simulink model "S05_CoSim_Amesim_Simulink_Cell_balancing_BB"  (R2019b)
settings: Solver=ode23s  StartTime=0  StopTime=25000  FixedStep=0.5  RelTol=1e-3  EnableMultiTasking=on
undefined symbols (not defined in the file): S05_CoSim_Amesim_Simulink_Cell_balancing
libraries: simulink x1
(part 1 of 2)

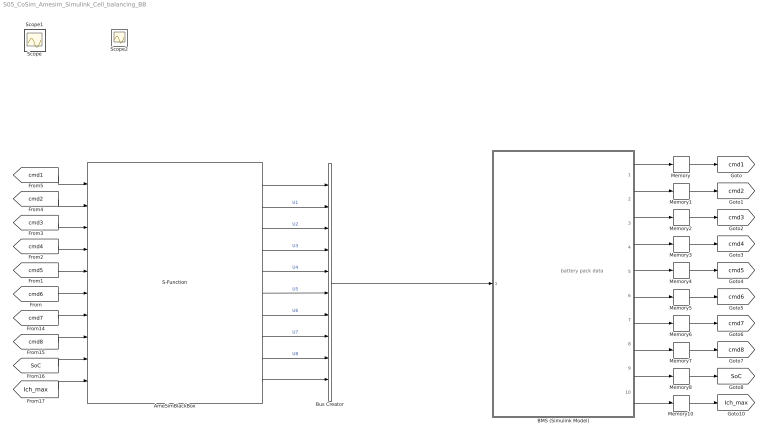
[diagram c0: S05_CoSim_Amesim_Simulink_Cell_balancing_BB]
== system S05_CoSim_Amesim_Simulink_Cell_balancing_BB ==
  note: battery pack data
  " BMS (Simulink Model)" : Subsystem
  AmeSimBlackBox : S-Function  InitFcn=clear S05_CoSim_Amesim_Simulink_Cell_balancing  StopFcn=clear S05_CoSim_Amesim_Simulink_Cell_balancing  FunctionName=S05_CoSim_Amesim_Simulink_Cell_balancing  Parameters=[0 0.01] [allrealparamnames] [allrealparamvalues] [allintparamnames] [allintparamvalues] [alltxtparamnames] [alltxtparamvalues]  SFunctionDeploymentMode=off  EnableBusSupport=off  mask(Simcenter Amesim S-function: S05_CoSim_Amesim_Simulink_Cell_balancing){IL_ns_paths=4, IL_SOCinit=90, IL_Cn=42, IL_Ichbalancing=8, IL_Idchbalancing=-8, IL_Tinit=23, IL_Tamb=23, IL_h_cell=222, IL_w_cell=211, IL_t_cell=12, IL_t_plate=1.5, IL_t_path=0.8, IL_w_path=2, IL_l_path=222, IL_DSOC1=3.46, IL_DSOC2=-4.33, IL_DSOC3=0.5, IL_DSOC4=0.38, IL_DSOC5=4.63, IL_DSOC6=-0.77, IL_DSOC7=2.73, IL_DSOC8=-1.36, IL_Ccoef1=1.033, IL_Ccoef2=1.053, IL_Ccoef3=0.953, IL_Ccoef4=1.058, IL_Ccoef5=0.926, IL_Ccoef6=1.064, IL_Ccoef7=0.956, IL_Ccoef8=1.077, IL_Rcoef1=0.93, IL_Rcoef2=0.876, IL_Rcoef3=1.029, IL_Rcoef4=0.863, IL_Rcoef5=0.85, IL_Rcoef6=1.044, IL_Rcoef7=0.878, IL_Rcoef8=1.146}
      mask prompts: IL_ns_paths "number of path per plate"; IL_SOCinit "inital state of charge"; IL_Cn "nominal capacity"; IL_Ichbalancing "balancing charge current"; IL_Idchbalancing "balancing discharge current"; IL_Tinit "initial temperature"; IL_Tamb "ambiant temperature"; IL_h_cell "height of the cell"; IL_w_cell "width of the cell"; IL_t_cell "thickness of the cell"; IL_t_plate "thickness of the plate"; IL_t_path "thickness of the coolant path"; IL_w_path "width of the coolant path"; IL_l_path "length of the coolant path"; IL_DSOC1 "SOC dispersion - cell 1"; IL_DSOC2 "SOC dispersion - cell 2"; IL_DSOC3 "SOC dispersion - cell 3"; IL_DSOC4 "SOC dispersion - cell 4"; IL_DSOC5 "SOC dispersion - cell 5"; IL_DSOC6 "SOC dispersion - cell 6"; IL_DSOC7 "SOC dispersion - cell 7"; IL_DSOC8 "SOC dispersion - cell 8"; IL_Ccoef1 "capacity dispersion coefficient - cell 1"; IL_Ccoef2 "capacity dispersion coefficient - cell 2"; IL_Ccoef3 "capacity dispersion coefficient - cell 3"; IL_Ccoef4 "capacity dispersion coefficient - cell 4"; IL_Ccoef5 "capacity dispersion coefficient - cell 5"; IL_Ccoef6 "capacity dispersion coefficient - cell 6"; IL_Ccoef7 "capacity dispersion coefficient - cell 7"; IL_Ccoef8 "capacity dispersion coefficient - cell 8"; IL_Rcoef1 "resistance dispersion coefficient - cell 1"; IL_Rcoef2 "resistance dispersion coefficient - cell 2"; IL_Rcoef3 "resistance dispersion coefficient - cell 3"; IL_Rcoef4 "resistance dispersion coefficient - cell 4"; IL_Rcoef5 "resistance dispersion coefficient - cell 5"; IL_Rcoef6 "resistance dispersion coefficient - cell 6"; IL_Rcoef7 "resistance dispersion coefficient- cell 7"; IL_Rcoef8 "resistance dispersion coefficient - cell 8"
      mask help: Mask for Simcenter Amesim to Simulink black-box.
      mask init:
      | allintparamnames=strvcat('ns_paths');allintparamvalues=[IL_ns_paths];allrealparamnames=strvcat('SOCinit','Cn','Ichbalancing','Idchbalancing','Tinit','Tamb','h_cell','w_cell','t_cell','t_plate','t_path','w_path','l_path','DSOC1','DSOC2','DSOC3','DSOC4','DSOC5','DSOC6','DSOC7','DSOC8','Ccoef1','Ccoef2','Ccoef3','Ccoef4','Ccoef5','Ccoef6','Ccoef7','Ccoef8','Rcoef1','Rcoef2','Rcoef3','Rcoef4','Rcoef5','Rcoef6','Rcoef7','Rcoef8');allrealparamvalues=[IL_SOCinit;IL_Cn;IL_Ichbalancing;IL_Idchbalancing;IL_Tinit;IL_Tamb;IL_h_cell;IL_w_cell;IL_t_cell;IL_t_plate;IL_t_path;IL_w_path;IL_l_path;IL_DSOC1;IL_DSOC2;IL_DSOC3;IL_DSOC4;IL_DSOC5;IL_DSOC6;IL_DSOC7;IL_DSOC8;IL_Ccoef1;IL_Ccoef2;IL_Ccoef3;IL_Ccoef4;IL_Ccoef5;IL_Ccoef6;IL_Ccoef7;IL_Ccoef8;IL_Rcoef1;IL_Rcoef2;IL_Rcoef3;IL_Rcoef4;IL_Rcoef5;IL_Rcoef6;IL_Rcoef7;IL_Rcoef8];alltxtparamnames=[];alltxtparamvalues=[];
  Bus Creator : BusCreator  Inputs=10
  Memory{,1..8,10} (10 alike) : Memory
  Scope : Scope
  Scope1 : Scope
  Scope2 : Scope
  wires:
  Memory/1 -> [cmd1]
  Memory2/1 -> [cmd3]
  Memory4/1 -> [cmd5]
  Memory3/1 -> [cmd4]
  Memory1/1 -> [cmd2]
  Memory5/1 -> [cmd6]
  Memory6/1 -> [cmd7]
  Memory7/1 -> [cmd8]
  Memory8/1 -> [SoC]
  AmeSimBlackBox/10 -> Bus Creator/10  "T"
  AmeSimBlackBox/9 -> Bus Creator/9  "U8"
  AmeSimBlackBox/7 -> Bus Creator/7  "U6"
  AmeSimBlackBox/6 -> Bus Creator/6  "U5"
  AmeSimBlackBox/5 -> Bus Creator/5  "U4"
  AmeSimBlackBox/4 -> Bus Creator/4  "U3"
  AmeSimBlackBox/3 -> Bus Creator/3  "U2"
  AmeSimBlackBox/2 -> Bus Creator/2  "U1"
  AmeSimBlackBox/8 -> Bus Creator/8  "U7"
  [cmd1] -> AmeSimBlackBox/1
  [cmd2] -> AmeSimBlackBox/2
  [cmd3] -> AmeSimBlackBox/3
  [cmd4] -> AmeSimBlackBox/4
  [cmd5] -> AmeSimBlackBox/5
  [cmd6] -> AmeSimBlackBox/6
  [cmd7] -> AmeSimBlackBox/7
  [cmd8] -> AmeSimBlackBox/8
  [SoC] -> AmeSimBlackBox/9
  AmeSimBlackBox/1 -> Bus Creator/1  "I"
  [Ich_max] -> AmeSimBlackBox/10
  Memory10/1 -> [Ich_max]
  Bus Creator/1 -> " BMS (Simulink Model)"/1(battery pack data)
  " BMS (Simulink Model)"/10(Ich_max) -> Memory10/1
  " BMS (Simulink Model)"/1(command cell1) -> Memory/1
  " BMS (Simulink Model)"/2(command cell2) -> Memory1/1
  " BMS (Simulink Model)"/3(command cell3) -> Memory2/1
  " BMS (Simulink Model)"/4(command cell4) -> Memory3/1
  " BMS (Simulink Model)"/5(command cell5) -> Memory4/1
  " BMS (Simulink Model)"/6(command cell6) -> Memory5/1
  " BMS (Simulink Model)"/7(command cell7) -> Memory6/1
  " BMS (Simulink Model)"/8(command cell8) -> Memory7/1
  " BMS (Simulink Model)"/9(mean SoC) -> Memory8/1

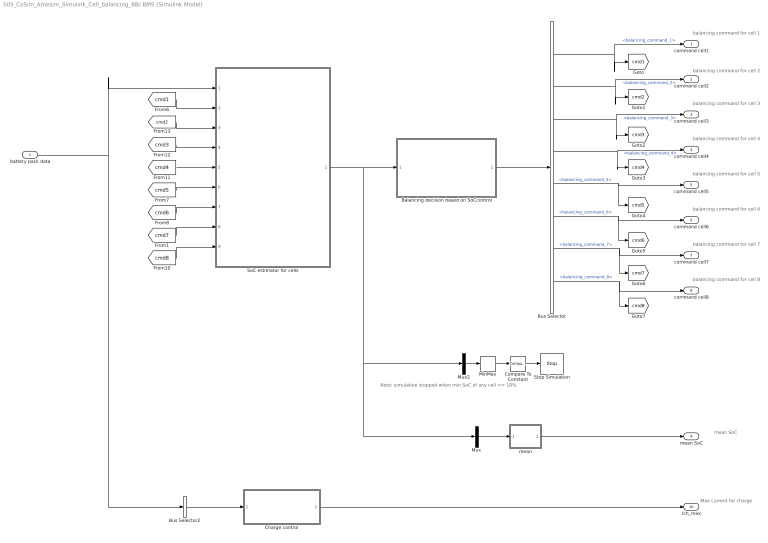
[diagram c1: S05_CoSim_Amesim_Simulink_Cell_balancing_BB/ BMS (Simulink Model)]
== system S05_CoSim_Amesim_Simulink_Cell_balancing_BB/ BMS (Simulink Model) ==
  note: balancing command for cell 1
  note: Max current for charge
  note: mean SoC
  note: Note: simulation stopped when min SoC of any cell <= 10%
  note: balancing command for cell 2
  note: balancing command for cell 3
  note: balancing command for cell 4
  note: balancing command for cell 5
  note: balancing command for cell 6
  note: balancing command for cell 7
  note: balancing command for cell 8
  battery pack data : Inport
  Balancing decision based on SoCcontrol : Subsystem
  Bus Selector : BusSelector  OutputSignals=balancing_command_1,balancing_command_2,balancing_command_3,balancing_command_4,balancing_command_5,balancing_command_6,balancing_command_7,balancing_command_8
  Bus Selector2 : BusSelector  OutputSignals=U1,U2,U3,U4,U5,U6,U7,U8  OutputAsBus=on
  Charge control : Subsystem
  Compare To Constant : simulink/Logic and Bit Operations/Compare To Constant  relop=<=  const=10  OutDataTypeStr=boolean
  MinMax : MinMax
  Mux : Mux  Inputs=1
  Mux2 : Mux  Inputs=1
  SoC estimator for cells : Subsystem
  Stop Simulation : Stop
  mean : MATLAB Function  TreatAsAtomicUnit=on
  command cell1 : Outport
  command cell2 : Outport  Port=2
  command cell3 : Outport  Port=3
  command cell4 : Outport  Port=4
  command cell5 : Outport  Port=5
  command cell6 : Outport  Port=6
  command cell7 : Outport  Port=7
  command cell8 : Outport  Port=8
  mean SoC : Outport  Port=9
  Ich_max : Outport  Port=10
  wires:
  Bus Selector/1 -> [cmd1], command cell1/1  "<balancing_command_1>"
  Bus Selector/6 -> [cmd6], command cell6/1  "<balancing_command_6>"
  Bus Selector/2 -> [cmd2], command cell2/1  "<balancing_command_2>"
  Bus Selector/5 -> [cmd5], command cell5/1  "<balancing_command_5>"
  Bus Selector/4 -> [cmd4], command cell4/1  "<balancing_command_4>"
  Bus Selector/3 -> [cmd3], command cell3/1  "<balancing_command_3>"
  Mux/1 -> mean/1(u)
  Bus Selector/8 -> [cmd8], command cell8/1  "<balancing_command_8>"
  mean/1(y) -> mean SoC/1
  Bus Selector/7 -> [cmd7], command cell7/1  "<balancing_command_7>"
  battery pack data/1 -> Bus Selector2/1, SoC estimator for cells/1(Battery pack data)
  Charge control/1(Ich_max) -> Ich_max/1
  Bus Selector2/1 -> Charge control/1(Ucells)
  Compare To Constant/1 -> Stop Simulation/1
  MinMax/1 -> Compare To Constant/1
  Mux2/1 -> MinMax/1
  Balancing decision based on SoCcontrol/1(balancing_commands) -> Bus Selector/1
  SoC estimator for cells/1(SoCs estimated of cells) -> Mux/1, Mux2/1, Balancing decision based on SoCcontrol/1(SOC_est)
  [cmd1] -> SoC estimator for cells/2(cmd_cell1)
  [cmd2] -> SoC estimator for cells/3(cmd_cell2)
  [cmd3] -> SoC estimator for cells/4(cmd_cell3)
  [cmd4] -> SoC estimator for cells/5(cmd_cell4)
  [cmd6] -> SoC estimator for cells/7(cmd_cell6)
  [cmd7] -> SoC estimator for cells/8(cmd_cell7)
  [cmd8] -> SoC estimator for cells/9(cmd_cell8)
  [cmd5] -> SoC estimator for cells/6(cmd_cell5)

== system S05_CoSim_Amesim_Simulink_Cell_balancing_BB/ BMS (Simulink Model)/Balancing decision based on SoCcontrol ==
  SOC_est : Inport
  Bus Creator1 : BusCreator  Inputs=8
  Bus Selector2 : BusSelector  OutputSignals=SOC1,SOC2,SOC3,SOC4,SOC5,SOC6,SOC7,SOC8
  Bus Selector3 : BusSelector  OutputSignals=SOC1,SOC2,SOC3,SOC4,SOC5,SOC6,SOC7,SOC8
  Mux : Mux  Inputs=8
  Subsystem1 : Subsystem
  Subsystem2 : Subsystem
  Subsystem3 : Subsystem
  Subsystem4 : Subsystem
  Subsystem5 : Subsystem
  Subsystem6 : Subsystem
  Subsystem7 : Subsystem
  Subsystem8 : Subsystem
  median : MATLAB Function  TreatAsAtomicUnit=on
  balancing_commands : Outport
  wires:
  Subsystem1/1(balancing_command) -> Bus Creator1/2  "balancing_command_2"
  Subsystem2/1(balancing_command) -> Bus Creator1/3  "balancing_command_3"
  Subsystem3/1(balancing_command) -> Bus Creator1/4  "balancing_command_4"
  Subsystem4/1(balancing_command) -> Bus Creator1/5  "balancing_command_5"
  Subsystem5/1(balancing_command) -> Bus Creator1/6  "balancing_command_6"
  median/1(y) -> Subsystem8/2(SOC_median), Subsystem7/2(SOC_median), Subsystem5/2(SOC_median), Subsystem4/2(SOC_median), Subsystem3/2(SOC_median), Subsystem2/2(SOC_median), Subsystem1/2(SOC_median), Subsystem6/2(SOC_median)
  Bus Selector2/1 -> Subsystem6/1(SOC_cell)  "<SOC1>"
  Subsystem6/1(balancing_command) -> Bus Creator1/1  "balancing_command_1"
  Bus Selector2/2 -> Subsystem1/1(SOC_cell)  "<SOC2>"
  Bus Selector2/3 -> Subsystem2/1(SOC_cell)  "<SOC3>"
  Bus Selector2/4 -> Subsystem3/1(SOC_cell)  "<SOC4>"
  Bus Selector2/5 -> Subsystem4/1(SOC_cell)  "<SOC5>"
  Bus Selector2/6 -> Subsystem5/1(SOC_cell)  "<SOC6>"
  SOC_est/1 -> Bus Selector3/1, Bus Selector2/1
  Bus Creator1/1 -> balancing_commands/1
  Bus Selector3/1 -> Mux/1  "<SOC1>"
  Bus Selector3/2 -> Mux/2  "<SOC2>"
  Bus Selector3/3 -> Mux/3  "<SOC3>"
  Bus Selector3/4 -> Mux/4  "<SOC4>"
  Bus Selector3/5 -> Mux/5  "<SOC5>"
  Bus Selector3/6 -> Mux/6  "<SOC6>"
  Mux/1 -> median/1(u)
  Bus Selector2/7 -> Subsystem7/1(SOC_cell)  "<SOC7>"
  Bus Selector2/8 -> Subsystem8/1(SOC_cell)  "<SOC8>"
  Subsystem7/1(balancing_command) -> Bus Creator1/7  "balancing_command_7"
  Subsystem8/1(balancing_command) -> Bus Creator1/8  "balancing_command_8"
  Bus Selector3/7 -> Mux/7  "<SOC7>"
  Bus Selector3/8 -> Mux/8  "<SOC8>"

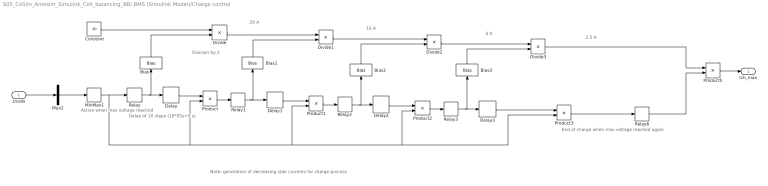
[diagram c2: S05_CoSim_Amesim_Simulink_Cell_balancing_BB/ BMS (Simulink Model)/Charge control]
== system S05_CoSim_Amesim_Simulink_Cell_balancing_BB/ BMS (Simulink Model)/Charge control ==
  note: Note: generation of decreasing stair currents for charge process
  note: Active when max voltage reached
  note: Delay of 10 steps (10*05s=5 s)
  note: 2.5 A
  note: 5 A
  note: 10 A
  note: 20 A
  note: Division by 2
  note: End of charge when max voltage reached again
  Ucells : Inport
  Bias{,1..3} (4 alike) : Bias  Bias=1
  Constant : Constant  Value=40
  Delay{,1..3} (4 alike) : Delay  DelayLength=10
  Divide{,1..3} (4 alike) : Product  Inputs=*/
  MinMax1 : MinMax  Function=max
  Mux2 : Mux  Inputs=1
  Product{,1..3,5} (5 alike) : Product
  Relay{,1..3} (4 alike) : Relay  OnSwitchValue=4.052  OffSwitchValue=4
  Relay6 : Relay  OnSwitchValue=4.052  OffSwitchValue=3.5  OnOutputValue=0  OffOutputValue=1
  Ich_max : Outport
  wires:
  Product3/1 -> Relay6/1
  Relay6/1 -> Product5/2
  Divide2/1 -> Divide3/1
  Product5/1 -> Ich_max/1
  Divide3/1 -> Product5/1
  Divide1/1 -> Divide2/1
  Relay3/1 -> Delay3/1, Bias3/1
  Product2/1 -> Relay3/1
  Bias2/1 -> Divide2/2
  Bias1/1 -> Divide1/2
  Relay1/1 -> Delay1/1, Bias1/1
  Bias3/1 -> Divide3/2
  Divide/1 -> Divide1/1
  MinMax1/1 -> Relay/1, Product3/2, Product2/2, Product1/2, Product/2
  Ucells/1 -> Mux2/1
  Mux2/1 -> MinMax1/1
  Relay/1 -> Delay/1, Bias/1
  Bias/1 -> Divide/2
  Constant/1 -> Divide/1
  Product/1 -> Relay1/1
  Product1/1 -> Relay2/1
  Delay/1 -> Product/1
  Delay1/1 -> Product1/1
  Delay2/1 -> Product2/1
  Delay3/1 -> Product3/1
  Relay2/1 -> Delay2/1, Bias2/1

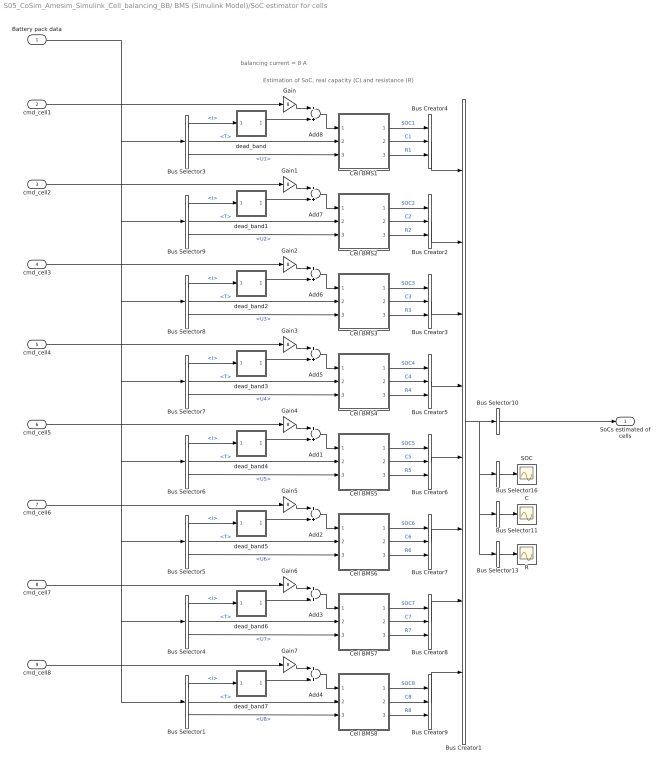
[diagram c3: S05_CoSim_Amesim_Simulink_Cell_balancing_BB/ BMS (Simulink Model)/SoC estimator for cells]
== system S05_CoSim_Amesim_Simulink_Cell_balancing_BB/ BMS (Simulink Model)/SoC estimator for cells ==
  note: Estimation of SoC, real capacity (C) and resistance (R)
  note: balancing current = 8 A
  Battery pack data : Inport
  cmd_cell1 : Inport  Port=2
  cmd_cell2 : Inport  Port=3
  cmd_cell3 : Inport  Port=4
  cmd_cell4 : Inport  Port=5
  cmd_cell5 : Inport  Port=6
  cmd_cell6 : Inport  Port=7
  cmd_cell7 : Inport  Port=8
  cmd_cell8 : Inport  Port=9
  Add{1..8} (8 alike) : Sum
  Bus Creator1 : BusCreator  Inputs=8
  Bus Creator{2..9} (8 alike) : BusCreator  Inputs=3
  Bus Selector1 : BusSelector  OutputSignals=I,T,U8
  Bus Selector10 : BusSelector  OutputSignals=signal1.SOC1,signal2.SOC2,signal3.SOC3,signal4.SOC4,signal5.SOC5,signal6.SOC6,signal7.SOC7,signal8.SOC8  OutputAsBus=on
  Bus Selector11 : BusSelector  OutputSignals=signal1.C1,signal2.C2,signal3.C3,signal4.C4,signal5.C5,signal6.C6,signal7.C7,signal8.C8  OutputAsBus=on
  Bus Selector13 : BusSelector  OutputSignals=signal1.R1,signal2.R2,signal3.R3,signal4.R4,signal5.R5,signal6.R6,signal7.R7,signal8.R8  OutputAsBus=on
  Bus Selector16 : BusSelector  OutputSignals=signal1.SOC1,signal2.SOC2,signal3.SOC3,signal4.SOC4,signal5.SOC5,signal6.SOC6,signal7.SOC7,signal8.SOC8  OutputAsBus=on
  Bus Selector3 : BusSelector  OutputSignals=I,T,U1
  Bus Selector4 : BusSelector  OutputSignals=I,T,U7
  Bus Selector5 : BusSelector  OutputSignals=I,T,U6
  Bus Selector6 : BusSelector  OutputSignals=I,T,U5
  Bus Selector7 : BusSelector  OutputSignals=I,T,U4
  Bus Selector8 : BusSelector  OutputSignals=I,T,U3
  Bus Selector9 : BusSelector  OutputSignals=I,T,U2
  C : Scope
  Cell BMS1 : Subsystem
  Cell BMS2 : Subsystem
  Cell BMS3 : Subsystem
  Cell BMS4 : Subsystem
  Cell BMS5 : Subsystem
  Cell BMS6 : Subsystem
  Cell BMS7 : Subsystem
  Cell BMS8 : Subsystem
  Gain{,1..7} (8 alike) : Gain  Gain=8
  R : Scope
  SOC : Scope
  dead_band : MATLAB Function  TreatAsAtomicUnit=on
  dead_band1 : MATLAB Function  TreatAsAtomicUnit=on
  dead_band2 : MATLAB Function  TreatAsAtomicUnit=on
  dead_band3 : MATLAB Function  TreatAsAtomicUnit=on
  dead_band4 : MATLAB Function  TreatAsAtomicUnit=on
  dead_band5 : MATLAB Function  TreatAsAtomicUnit=on
  dead_band6 : MATLAB Function  TreatAsAtomicUnit=on
  dead_band7 : MATLAB Function  TreatAsAtomicUnit=on
  SoCs estimated of cells : Outport
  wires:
  cmd_cell7/1 -> Gain6/1
  Gain5/1 -> Add2/1
  Bus Creator1/1 -> Bus Selector10/1, Bus Selector16/1, Bus Selector13/1, Bus Selector11/1
  Bus Creator9/1 -> Bus Creator1/8
  Cell BMS7/1(SOC) -> Bus Creator8/1  "SOC7"
  Bus Creator5/1 -> Bus Creator1/4
  Cell BMS8/1(SOC) -> Bus Creator9/1  "SOC8"
  Bus Creator3/1 -> Bus Creator1/3
  Cell BMS5/3(R) -> Bus Creator6/3  "R5"
  Cell BMS3/1(SOC) -> Bus Creator3/1  "SOC3"
  Bus Selector13/1 -> R/1
  Cell BMS4/3(R) -> Bus Creator5/3  "R4"
  Add1/1 -> Cell BMS5/1(I)
  cmd_cell3/1 -> Gain2/1
  Gain/1 -> Add8/1
  Gain3/1 -> Add5/1
  cmd_cell8/1 -> Gain7/1
  cmd_cell5/1 -> Gain4/1
  cmd_cell4/1 -> Gain3/1
  Add2/1 -> Cell BMS6/1(I)
  Gain2/1 -> Add6/1
  Gain1/1 -> Add7/1
  cmd_cell2/1 -> Gain1/1
  Bus Selector16/1 -> SOC/1
  Bus Selector10/1 -> SoCs estimated of cells/1
  Bus Selector11/1 -> C/1
  Cell BMS6/3(R) -> Bus Creator7/3  "R6"
  Cell BMS3/3(R) -> Bus Creator3/3  "R3"
  cmd_cell1/1 -> Gain/1
  Bus Selector3/3 -> Cell BMS1/3(U)  "<U1>"
  Bus Selector1/2 -> Cell BMS8/2(Temp)  "<T>"
  Bus Selector1/3 -> Cell BMS8/3(U)  "<U8>"
  Add8/1 -> Cell BMS1/1(I)
  Bus Selector3/2 -> Cell BMS1/2(Temp)  "<T>"
  Cell BMS3/2(C) -> Bus Creator3/2  "C3"
  Bus Selector1/1 -> dead_band7/1(u)  "<I>"
  Bus Selector4/1 -> dead_band6/1(u)  "<I>"
  Bus Selector7/3 -> Cell BMS4/3(U)  "<U4>"
  Bus Selector5/3 -> Cell BMS6/3(U)  "<U6>"
  Add6/1 -> Cell BMS3/1(I)
  Cell BMS1/3(R) -> Bus Creator4/3  "R1"
  Bus Selector5/2 -> Cell BMS6/2(Temp)  "<T>"
  Bus Selector6/2 -> Cell BMS5/2(Temp)  "<T>"
  Bus Selector9/2 -> Cell BMS2/2(Temp)  "<T>"
  Bus Selector4/2 -> Cell BMS7/2(Temp)  "<T>"
  Add5/1 -> Cell BMS4/1(I)
  Bus Selector7/1 -> dead_band3/1(u)  "<I>"
  Bus Selector5/1 -> dead_band5/1(u)  "<I>"
  Bus Selector4/3 -> Cell BMS7/3(U)  "<U7>"
  Bus Selector6/3 -> Cell BMS5/3(U)  "<U5>"
  Bus Selector8/3 -> Cell BMS3/3(U)  "<U3>"
  Bus Selector7/2 -> Cell BMS4/2(Temp)  "<T>"
  Bus Selector8/1 -> dead_band2/1(u)  "<I>"
  Bus Selector8/2 -> Cell BMS3/2(Temp)  "<T>"
  Bus Selector9/1 -> dead_band1/1(u)  "<I>"
  Cell BMS1/1(SOC) -> Bus Creator4/1  "SOC1"
  Bus Selector9/3 -> Cell BMS2/3(U)  "<U2>"
  Add7/1 -> Cell BMS2/1(I)
  Bus Creator2/1 -> Bus Creator1/2
  Cell BMS2/1(SOC) -> Bus Creator2/1  "SOC2"
  Bus Selector6/1 -> dead_band4/1(u)  "<I>"
  Cell BMS2/3(R) -> Bus Creator2/3  "R2"
  Cell BMS2/2(C) -> Bus Creator2/2  "C2"
  Cell BMS5/1(SOC) -> Bus Creator6/1  "SOC5"
  Cell BMS7/2(C) -> Bus Creator8/2  "C7"
  Cell BMS4/1(SOC) -> Bus Creator5/1  "SOC4"
  Bus Creator6/1 -> Bus Creator1/5
  Cell BMS1/2(C) -> Bus Creator4/2  "C1"
  Bus Creator4/1 -> Bus Creator1/1
  Cell BMS8/3(R) -> Bus Creator9/3  "R8"
  Cell BMS6/1(SOC) -> Bus Creator7/1  "SOC6"
  Cell BMS7/3(R) -> Bus Creator8/3  "R7"
  Cell BMS4/2(C) -> Bus Creator5/2  "C4"
  Cell BMS5/2(C) -> Bus Creator6/2  "C5"
  Bus Creator8/1 -> Bus Creator1/7
  Cell BMS6/2(C) -> Bus Creator7/2  "C6"
  Cell BMS8/2(C) -> Bus Creator9/2  "C8"
  Bus Creator7/1 -> Bus Creator1/6
  Gain6/1 -> Add3/1
  cmd_cell6/1 -> Gain5/1
  Add3/1 -> Cell BMS7/1(I)
  Gain4/1 -> Add1/1
  Add4/1 -> Cell BMS8/1(I)
  Gain7/1 -> Add4/1
  Battery pack data/1 -> Bus Selector1/1, Bus Selector4/1, Bus Selector5/1, Bus Selector6/1, Bus Selector7/1, Bus Selector8/1, Bus Selector9/1, Bus Selector3/1
  dead_band/1(y) -> Add8/2
  Bus Selector3/1 -> dead_band/1(u)  "<I>"
  dead_band1/1(y) -> Add7/2
  dead_band2/1(y) -> Add6/2
  dead_band3/1(y) -> Add5/2
  dead_band4/1(y) -> Add1/2
  dead_band5/1(y) -> Add2/2
  dead_band6/1(y) -> Add3/2
  dead_band7/1(y) -> Add4/2

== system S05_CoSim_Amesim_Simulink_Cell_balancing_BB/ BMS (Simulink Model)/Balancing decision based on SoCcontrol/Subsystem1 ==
  SOC_cell : Inport
  SOC_median : Inport  Port=2
  Add1 : Sum  Inputs=+-
  Add2 : Sum
  Relay : Relay  OnSwitchValue=0.3  OffSwitchValue=0.0  OnOutputValue=-1
  Relay1 : Relay  OnSwitchValue=0.0  OffSwitchValue=-0.3  OnOutputValue=0  OffOutputValue=1
  balancing_command : Outport
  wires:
  SOC_cell/1 -> Add1/1
  SOC_median/1 -> Add1/2
  Add1/1 -> Relay1/1, Relay/1
  Relay1/1 -> Add2/2
  Relay/1 -> Add2/1
  Add2/1 -> balancing_command/1

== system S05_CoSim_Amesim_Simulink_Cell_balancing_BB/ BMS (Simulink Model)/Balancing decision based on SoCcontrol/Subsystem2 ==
  SOC_cell : Inport
  SOC_median : Inport  Port=2
  Add1 : Sum  Inputs=+-
  Add2 : Sum
  Relay : Relay  OnSwitchValue=0.3  OffSwitchValue=0.0  OnOutputValue=-1
  Relay1 : Relay  OnSwitchValue=0.0  OffSwitchValue=-0.3  OnOutputValue=0  OffOutputValue=1
  balancing_command : Outport
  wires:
  SOC_cell/1 -> Add1/1
  SOC_median/1 -> Add1/2
  Add1/1 -> Relay1/1, Relay/1
  Relay1/1 -> Add2/2
  Relay/1 -> Add2/1
  Add2/1 -> balancing_command/1

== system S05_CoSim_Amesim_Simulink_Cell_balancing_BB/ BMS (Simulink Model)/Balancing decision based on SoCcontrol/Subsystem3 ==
  SOC_cell : Inport
  SOC_median : Inport  Port=2
  Add1 : Sum  Inputs=+-
  Add2 : Sum
  Relay : Relay  OnSwitchValue=0.3  OffSwitchValue=0.0  OnOutputValue=-1
  Relay1 : Relay  OnSwitchValue=0.0  OffSwitchValue=-0.3  OnOutputValue=0  OffOutputValue=1
  balancing_command : Outport
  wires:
  SOC_cell/1 -> Add1/1
  SOC_median/1 -> Add1/2
  Add1/1 -> Relay1/1, Relay/1
  Relay1/1 -> Add2/2
  Relay/1 -> Add2/1
  Add2/1 -> balancing_command/1

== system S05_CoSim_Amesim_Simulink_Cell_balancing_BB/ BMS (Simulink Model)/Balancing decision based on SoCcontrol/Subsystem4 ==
  SOC_cell : Inport
  SOC_median : Inport  Port=2
  Add1 : Sum  Inputs=+-
  Add2 : Sum
  Relay : Relay  OnSwitchValue=0.3  OffSwitchValue=0.0  OnOutputValue=-1
  Relay1 : Relay  OnSwitchValue=0.0  OffSwitchValue=-0.3  OnOutputValue=0  OffOutputValue=1
  balancing_command : Outport
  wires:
  SOC_cell/1 -> Add1/1
  SOC_median/1 -> Add1/2
  Add1/1 -> Relay1/1, Relay/1
  Relay1/1 -> Add2/2
  Relay/1 -> Add2/1
  Add2/1 -> balancing_command/1

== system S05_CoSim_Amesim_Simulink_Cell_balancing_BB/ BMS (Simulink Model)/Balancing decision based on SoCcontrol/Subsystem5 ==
  SOC_cell : Inport
  SOC_median : Inport  Port=2
  Add1 : Sum  Inputs=+-
  Add2 : Sum
  Relay : Relay  OnSwitchValue=0.3  OffSwitchValue=0.0  OnOutputValue=-1
  Relay1 : Relay  OnSwitchValue=0.0  OffSwitchValue=-0.3  OnOutputValue=0  OffOutputValue=1
  balancing_command : Outport
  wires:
  SOC_cell/1 -> Add1/1
  SOC_median/1 -> Add1/2
  Add1/1 -> Relay1/1, Relay/1
  Relay1/1 -> Add2/2
  Relay/1 -> Add2/1
  Add2/1 -> balancing_command/1

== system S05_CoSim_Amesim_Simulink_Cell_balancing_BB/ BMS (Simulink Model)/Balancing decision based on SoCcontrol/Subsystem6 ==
  SOC_cell : Inport
  SOC_median : Inport  Port=2
  Add1 : Sum  Inputs=+-
  Add2 : Sum
  Relay : Relay  OnSwitchValue=0.3  OffSwitchValue=0.0  OnOutputValue=-1
  Relay1 : Relay  OnSwitchValue=0.0  OffSwitchValue=-0.3  OnOutputValue=0  OffOutputValue=1
  balancing_command : Outport
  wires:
  SOC_cell/1 -> Add1/1
  SOC_median/1 -> Add1/2
  Add1/1 -> Relay1/1, Relay/1
  Relay1/1 -> Add2/2
  Relay/1 -> Add2/1
  Add2/1 -> balancing_command/1

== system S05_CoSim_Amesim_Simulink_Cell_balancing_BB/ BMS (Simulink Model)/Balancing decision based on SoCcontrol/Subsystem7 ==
  SOC_cell : Inport
  SOC_median : Inport  Port=2
  Add1 : Sum  Inputs=+-
  Add2 : Sum
  Relay : Relay  OnSwitchValue=0.3  OffSwitchValue=0.0  OnOutputValue=-1
  Relay1 : Relay  OnSwitchValue=0.0  OffSwitchValue=-0.3  OnOutputValue=0  OffOutputValue=1
  balancing_command : Outport
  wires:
  SOC_cell/1 -> Add1/1
  SOC_median/1 -> Add1/2
  Add1/1 -> Relay1/1, Relay/1
  Relay1/1 -> Add2/2
  Relay/1 -> Add2/1
  Add2/1 -> balancing_command/1

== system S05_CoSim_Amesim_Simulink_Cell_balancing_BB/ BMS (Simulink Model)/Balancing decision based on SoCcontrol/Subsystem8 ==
  SOC_cell : Inport
  SOC_median : Inport  Port=2
  Add1 : Sum  Inputs=+-
  Add2 : Sum
  Relay : Relay  OnSwitchValue=0.3  OffSwitchValue=0.0  OnOutputValue=-1
  Relay1 : Relay  OnSwitchValue=0.0  OffSwitchValue=-0.3  OnOutputValue=0  OffOutputValue=1
  balancing_command : Outport
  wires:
  SOC_cell/1 -> Add1/1
  SOC_median/1 -> Add1/2
  Add1/1 -> Relay1/1, Relay/1
  Relay1/1 -> Add2/2
  Relay/1 -> Add2/1
  Add2/1 -> balancing_command/1

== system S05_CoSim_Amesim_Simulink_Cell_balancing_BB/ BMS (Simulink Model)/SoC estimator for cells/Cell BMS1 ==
  note: Temperature
  I : Inport
  Temp : Inport  Port=2
  U : Inport  Port=3
  SOC estimator : Subsystem  mask{SOC_init=90, Cnom=42, gainU=50}
      mask prompts: SOC_init "inital state of charge"; Cnom "nominal capacity"; gainU "gain for voltage translation"
  SOH identification : Subsystem
  voltage translation weight : Subsystem
  SOC : Outport
  C : Outport  Port=2
  R : Outport  Port=3
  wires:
  SOC estimator/1(SOC) -> SOC/1
  SOH identification/1(C) -> C/1, SOC estimator/5(C)
  SOC estimator/2(Uerror) -> SOH identification/3(Urerror)
  SOC estimator/3(Icorrect) -> SOH identification/4(Icorrect)
  SOH identification/2(R) -> R/1, SOC estimator/6(R)
  U/1 -> SOC estimator/4(U)
  Temp/1 -> SOC estimator/3(Temp)
  I/1 -> voltage translation weight/1(I), SOC estimator/1(I), SOH identification/1(I)
  voltage translation weight/1(VTweight) -> SOH identification/2(VTweight), SOC estimator/2(VTweight)

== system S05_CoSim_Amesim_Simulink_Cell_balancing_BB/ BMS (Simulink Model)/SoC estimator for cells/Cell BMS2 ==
  I : Inport
  Temp : Inport  Port=2
  U : Inport  Port=3
  SOC estimator : Subsystem  mask{SOC_init=90, Cnom=42, gainU=50}
      mask prompts: SOC_init "inital state of charge"; Cnom "nominal capacity"; gainU "gain for voltage translation"
  SOH identification : Subsystem
  voltage translation weight : Subsystem
  SOC : Outport
  C : Outport  Port=2
  R : Outport  Port=3
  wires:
  SOC estimator/1(SOC) -> SOC/1
  SOH identification/1(C) -> C/1, SOC estimator/5(C)
  SOC estimator/2(Uerror) -> SOH identification/3(Urerror)
  SOC estimator/3(Icorrect) -> SOH identification/4(Icorrect)
  SOH identification/2(R) -> R/1, SOC estimator/6(R)
  U/1 -> SOC estimator/4(U)
  Temp/1 -> SOC estimator/3(Temp)
  I/1 -> voltage translation weight/1(I), SOC estimator/1(I), SOH identification/1(I)
  voltage translation weight/1(VTweight) -> SOH identification/2(VTweight), SOC estimator/2(VTweight)

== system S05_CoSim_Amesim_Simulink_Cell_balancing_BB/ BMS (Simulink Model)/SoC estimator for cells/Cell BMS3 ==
  I : Inport
  Temp : Inport  Port=2
  U : Inport  Port=3
  SOC estimator : Subsystem  mask{SOC_init=90, Cnom=42, gainU=50}
      mask prompts: SOC_init "inital state of charge"; Cnom "nominal capacity"; gainU "gain for voltage translation"
  SOH identification : Subsystem
  voltage translation weight : Subsystem
  SOC : Outport
  C : Outport  Port=2
  R : Outport  Port=3
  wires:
  SOC estimator/1(SOC) -> SOC/1
  SOH identification/1(C) -> C/1, SOC estimator/5(C)
  SOC estimator/2(Uerror) -> SOH identification/3(Urerror)
  SOC estimator/3(Icorrect) -> SOH identification/4(Icorrect)
  SOH identification/2(R) -> R/1, SOC estimator/6(R)
  U/1 -> SOC estimator/4(U)
  Temp/1 -> SOC estimator/3(Temp)
  I/1 -> voltage translation weight/1(I), SOC estimator/1(I), SOH identification/1(I)
  voltage translation weight/1(VTweight) -> SOH identification/2(VTweight), SOC estimator/2(VTweight)

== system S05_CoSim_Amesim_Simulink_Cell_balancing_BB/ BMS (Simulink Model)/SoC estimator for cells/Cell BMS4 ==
  I : Inport
  Temp : Inport  Port=2
  U : Inport  Port=3
  SOC estimator : Subsystem  mask{SOC_init=90, Cnom=42, gainU=50}
      mask prompts: SOC_init "inital state of charge"; Cnom "nominal capacity"; gainU "gain for voltage translation"
  SOH identification : Subsystem
  voltage translation weight : Subsystem
  SOC : Outport
  C : Outport  Port=2
  R : Outport  Port=3
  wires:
  SOC estimator/1(SOC) -> SOC/1
  SOH identification/1(C) -> C/1, SOC estimator/5(C)
  SOC estimator/2(Uerror) -> SOH identification/3(Urerror)
  SOC estimator/3(Icorrect) -> SOH identification/4(Icorrect)
  SOH identification/2(R) -> R/1, SOC estimator/6(R)
  U/1 -> SOC estimator/4(U)
  Temp/1 -> SOC estimator/3(Temp)
  I/1 -> voltage translation weight/1(I), SOC estimator/1(I), SOH identification/1(I)
  voltage translation weight/1(VTweight) -> SOH identification/2(VTweight), SOC estimator/2(VTweight)

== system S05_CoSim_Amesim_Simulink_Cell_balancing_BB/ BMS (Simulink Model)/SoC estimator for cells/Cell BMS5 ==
  I : Inport
  Temp : Inport  Port=2
  U : Inport  Port=3
  SOC estimator : Subsystem  mask{SOC_init=90, Cnom=42, gainU=50}
      mask prompts: SOC_init "inital state of charge"; Cnom "nominal capacity"; gainU "gain for voltage translation"
  SOH identification : Subsystem
  voltage translation weight : Subsystem
  SOC : Outport
  C : Outport  Port=2
  R : Outport  Port=3
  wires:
  SOC estimator/1(SOC) -> SOC/1
  SOH identification/1(C) -> C/1, SOC estimator/5(C)
  SOC estimator/2(Uerror) -> SOH identification/3(Urerror)
  SOC estimator/3(Icorrect) -> SOH identification/4(Icorrect)
  SOH identification/2(R) -> R/1, SOC estimator/6(R)
  U/1 -> SOC estimator/4(U)
  Temp/1 -> SOC estimator/3(Temp)
  I/1 -> voltage translation weight/1(I), SOC estimator/1(I), SOH identification/1(I)
  voltage translation weight/1(VTweight) -> SOH identification/2(VTweight), SOC estimator/2(VTweight)

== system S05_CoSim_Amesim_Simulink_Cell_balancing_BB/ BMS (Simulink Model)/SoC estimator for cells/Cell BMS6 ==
  I : Inport
  Temp : Inport  Port=2
  U : Inport  Port=3
  SOC estimator : Subsystem  mask{SOC_init=90, Cnom=42, gainU=50}
      mask prompts: SOC_init "inital state of charge"; Cnom "nominal capacity"; gainU "gain for voltage translation"
  SOH identification : Subsystem
  voltage translation weight : Subsystem
  SOC : Outport
  C : Outport  Port=2
  R : Outport  Port=3
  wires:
  SOC estimator/1(SOC) -> SOC/1
  SOH identification/1(C) -> C/1, SOC estimator/5(C)
  SOC estimator/2(Uerror) -> SOH identification/3(Urerror)
  SOC estimator/3(Icorrect) -> SOH identification/4(Icorrect)
  SOH identification/2(R) -> R/1, SOC estimator/6(R)
  U/1 -> SOC estimator/4(U)
  Temp/1 -> SOC estimator/3(Temp)
  I/1 -> voltage translation weight/1(I), SOC estimator/1(I), SOH identification/1(I)
  voltage translation weight/1(VTweight) -> SOH identification/2(VTweight), SOC estimator/2(VTweight)

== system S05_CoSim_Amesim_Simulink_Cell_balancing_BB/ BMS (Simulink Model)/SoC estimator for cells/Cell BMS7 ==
  I : Inport
  Temp : Inport  Port=2
  U : Inport  Port=3
  SOC estimator : Subsystem  mask{SOC_init=90, Cnom=42, gainU=50}
      mask prompts: SOC_init "inital state of charge"; Cnom "nominal capacity"; gainU "gain for voltage translation"
  SOH identification : Subsystem
  voltage translation weight : Subsystem
  SOC : Outport
  C : Outport  Port=2
  R : Outport  Port=3
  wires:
  SOC estimator/1(SOC) -> SOC/1
  SOH identification/1(C) -> C/1, SOC estimator/5(C)
  SOC estimator/2(Uerror) -> SOH identification/3(Urerror)
  SOC estimator/3(Icorrect) -> SOH identification/4(Icorrect)
  SOH identification/2(R) -> R/1, SOC estimator/6(R)
  U/1 -> SOC estimator/4(U)
  Temp/1 -> SOC estimator/3(Temp)
  I/1 -> voltage translation weight/1(I), SOC estimator/1(I), SOH identification/1(I)
  voltage translation weight/1(VTweight) -> SOH identification/2(VTweight), SOC estimator/2(VTweight)

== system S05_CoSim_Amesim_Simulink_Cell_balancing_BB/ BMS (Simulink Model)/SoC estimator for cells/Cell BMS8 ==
  I : Inport
  Temp : Inport  Port=2
  U : Inport  Port=3
  SOC estimator : Subsystem  mask{SOC_init=90, Cnom=42, gainU=50}
      mask prompts: SOC_init "inital state of charge"; Cnom "nominal capacity"; gainU "gain for voltage translation"
  SOH identification : Subsystem
  voltage translation weight : Subsystem
  SOC : Outport
  C : Outport  Port=2
  R : Outport  Port=3
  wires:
  SOC estimator/1(SOC) -> SOC/1
  SOH identification/1(C) -> C/1, SOC estimator/5(C)
  SOC estimator/2(Uerror) -> SOH identification/3(Urerror)
  SOC estimator/3(Icorrect) -> SOH identification/4(Icorrect)
  SOH identification/2(R) -> R/1, SOC estimator/6(R)
  U/1 -> SOC estimator/4(U)
  Temp/1 -> SOC estimator/3(Temp)
  I/1 -> voltage translation weight/1(I), SOC estimator/1(I), SOH identification/1(I)
  voltage translation weight/1(VTweight) -> SOH identification/2(VTweight), SOC estimator/2(VTweight)

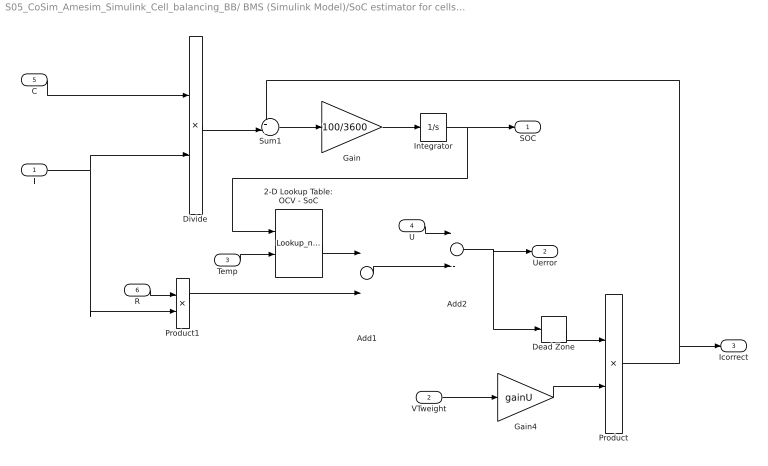
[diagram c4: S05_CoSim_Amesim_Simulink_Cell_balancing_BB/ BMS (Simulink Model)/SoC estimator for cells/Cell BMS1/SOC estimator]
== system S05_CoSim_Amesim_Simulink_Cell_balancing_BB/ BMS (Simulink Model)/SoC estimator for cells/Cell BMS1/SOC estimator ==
  I : Inport
  VTweight : Inport  Port=2
  Temp : Inport  Port=3
  U : Inport  Port=4
  C : Inport  Port=5
  R : Inport  Port=6
  2-D Lookup Table: OCV - SoC : Lookup_n-D  BreakpointsForDimension1=[0, 5, 10, 15, 20, 25, 30, 35, 40, 45, 50, 55, 60, 65, 70, 75, 80, 85, 90, 95, 100]  BreakpointsForDimension2=[0.00, 23.00, 40.00]  Table=[3.00912, 3.025112, 3.036932; 3.332236, 3.339581, 3.34501; 3.459481, 3.463587, 3.466622; 3.495249, 3.49837, 3.500677; 3.531047, 3.53332, 3.535; 3.560502, 3.562569, 3.564097; 3.588662, 3.589579, 3.590256; 3.62715, 3.625996, 3.625143; 3.648255, 3.64543, 3.643341; 3.66652, 3.663455, 3.66119; 3.685242, 3.681938, 3.679495; 3.70967, 3.706246, 3.703715; 3.738426, 3.735163, 3.732751; 3.780458, 3.777286, 3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  InternalRulePriority=Speed  RndMeth=Simplest
  Add1 : Sum
  Add2 : Sum  Inputs=+-
  Dead Zone : DeadZone  LowerValue=-0.005  UpperValue=0.005
  Divide : Product  Inputs=/*
  Gain : Gain  Gain=100/3600
  Gain4 : Gain  Gain=gainU
  Integrator : Integrator  InitialCondition=SOC_init
  Product : Product
  Product1 : Product
  Sum1 : Sum  Inputs=++|
  SOC : Outport
  Uerror : Outport  Port=2
  Icorrect : Outport  Port=3
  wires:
  Integrator/1 -> SOC/1, 2-D Lookup Table: OCV - SoC/1
  Gain/1 -> Integrator/1
  Sum1/1 -> Gain/1
  Add2/1 -> Uerror/1, Dead Zone/1
  Temp/1 -> 2-D Lookup Table: OCV - SoC/2
  C/1 -> Divide/1
  Divide/1 -> Sum1/2
  Gain4/1 -> Product/2
  R/1 -> Product1/1
  2-D Lookup Table: OCV - SoC/1 -> Add1/1
  Add1/1 -> Add2/2
  U/1 -> Add2/1
  Product1/1 -> Add1/2
  I/1 -> Divide/2, Product1/2
  Dead Zone/1 -> Product/1
  Product/1 -> Icorrect/1, Sum1/1
  VTweight/1 -> Gain4/1

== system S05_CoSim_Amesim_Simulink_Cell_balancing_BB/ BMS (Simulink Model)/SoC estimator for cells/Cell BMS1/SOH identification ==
  note: Resistance estimation (ohm)
  note: Capacity estimation (Ah)
  I : Inport
  VTweight : Inport  Port=2
  Urerror : Inport  Port=3
  Icorrect : Inport  Port=4
  Cnom : Constant  Value=42
  Divide : Product  Inputs=**
  Divide1 : Product  Inputs=**
  Integrator3 : Integrator
  Integrator6 : Integrator
  Math Function : Math
  Math Function1 : Math
  Rnom : Constant  Value=0.0022
  Subsystem : Subsystem
  Subsystem6 : Subsystem
  C : Outport
  R : Outport  Port=2
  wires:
  I/1 -> Subsystem6/1(I), Subsystem/1(I)
  Rnom/1 -> Divide1/1
  Divide1/1 -> R/1
  Divide/1 -> C/1
  Subsystem6/1(dCcoef) -> Integrator6/1
  Integrator6/1 -> Math Function/1
  Icorrect/1 -> Subsystem6/3(Icorrect)
  Cnom/1 -> Divide/1
  Urerror/1 -> Subsystem/2(Uerror)
  Subsystem/1(dRcoef) -> Integrator3/1
  Integrator3/1 -> Math Function1/1
  VTweight/1 -> Subsystem6/2(VTweight)
  Math Function/1 -> Divide/2
  Math Function1/1 -> Divide1/2

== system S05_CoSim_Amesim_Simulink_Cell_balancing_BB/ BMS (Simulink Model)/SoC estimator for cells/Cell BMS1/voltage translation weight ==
  I : Inport
  1-D Lookup Table : Lookup_n-D  NumberOfTableDimensions=1  BreakpointsForDimension1=[-0.6,-0.5,-0.1,0,0.1,0.5,0.6]  Table=[0,0,0.2,1,0.2,0,0]  InternalRulePriority=Speed  RndMeth=Simplest
  Add3 : Sum
  Gain2 : Gain  Gain=1/42
  Gain3 : Gain  Gain=0.5
  Transfer Fcn1 : TransferFcn  Denominator=[20*20*20 3*20*20 3*20 1]
  abs : Fcn  Expr=abs(u(1))
  VTweight : Outport
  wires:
  abs/1 -> Transfer Fcn1/1, Add3/1
  Gain2/1 -> abs/1  "Crate"
  Transfer Fcn1/1 -> Add3/2
  Add3/1 -> Gain3/1
  Gain3/1 -> 1-D Lookup Table/1
  I/1 -> Gain2/1
  1-D Lookup Table/1 -> VTweight/1

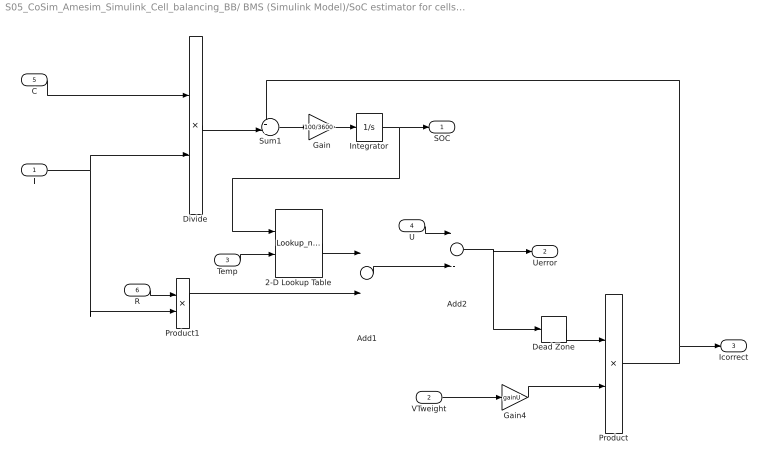
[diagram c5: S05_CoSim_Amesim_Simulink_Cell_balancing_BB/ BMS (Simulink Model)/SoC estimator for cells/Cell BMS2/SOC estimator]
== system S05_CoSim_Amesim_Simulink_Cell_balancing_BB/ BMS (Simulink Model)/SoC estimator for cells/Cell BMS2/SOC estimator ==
  I : Inport
  VTweight : Inport  Port=2
  Temp : Inport  Port=3
  U : Inport  Port=4
  C : Inport  Port=5
  R : Inport  Port=6
  2-D Lookup Table : Lookup_n-D  BreakpointsForDimension1=[0, 5, 10, 15, 20, 25, 30, 35, 40, 45, 50, 55, 60, 65, 70, 75, 80, 85, 90, 95, 100]  BreakpointsForDimension2=[0.00, 23.00, 40.00]  Table=[3.00912, 3.025112, 3.036932; 3.332236, 3.339581, 3.34501; 3.459481, 3.463587, 3.466622; 3.495249, 3.49837, 3.500677; 3.531047, 3.53332, 3.535; 3.560502, 3.562569, 3.564097; 3.588662, 3.589579, 3.590256; 3.62715, 3.625996, 3.625143; 3.648255, 3.64543, 3.643341; 3.66652, 3.663455, 3.66119; 3.685242, 3.681938, 3.679495; 3.70967, 3.706246, 3.703715; 3.738426, 3.735163, 3.732751; 3.780458, 3.777286, 3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  InternalRulePriority=Speed  RndMeth=Simplest
  Add1 : Sum
  Add2 : Sum  Inputs=+-
  Dead Zone : DeadZone  LowerValue=-0.005  UpperValue=0.005
  Divide : Product  Inputs=/*
  Gain : Gain  Gain=100/3600
  Gain4 : Gain  Gain=gainU
  Integrator : Integrator  InitialCondition=SOC_init
  Product : Product
  Product1 : Product
  Sum1 : Sum  Inputs=++|
  SOC : Outport
  Uerror : Outport  Port=2
  Icorrect : Outport  Port=3
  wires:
  Integrator/1 -> SOC/1, 2-D Lookup Table/1
  Gain/1 -> Integrator/1
  Sum1/1 -> Gain/1
  Add2/1 -> Uerror/1, Dead Zone/1
  Temp/1 -> 2-D Lookup Table/2
  C/1 -> Divide/1
  Divide/1 -> Sum1/2
  Gain4/1 -> Product/2
  R/1 -> Product1/1
  2-D Lookup Table/1 -> Add1/1
  Add1/1 -> Add2/2
  U/1 -> Add2/1
  Product1/1 -> Add1/2
  I/1 -> Divide/2, Product1/2
  Dead Zone/1 -> Product/1
  Product/1 -> Icorrect/1, Sum1/1
  VTweight/1 -> Gain4/1

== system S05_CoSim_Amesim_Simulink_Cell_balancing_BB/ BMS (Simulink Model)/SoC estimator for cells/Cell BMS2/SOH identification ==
  I : Inport
  VTweight : Inport  Port=2
  Urerror : Inport  Port=3
  Icorrect : Inport  Port=4
  Cnom : Constant  Value=42
  Divide : Product  Inputs=**
  Divide1 : Product  Inputs=**
  Integrator3 : Integrator
  Integrator6 : Integrator
  Math Function : Math
  Math Function1 : Math
  Rnom : Constant  Value=0.0022
  Subsystem : Subsystem
  Subsystem6 : Subsystem
  C : Outport
  R : Outport  Port=2
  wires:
  I/1 -> Subsystem6/1(I), Subsystem/1(I)
  Rnom/1 -> Divide1/1
  Divide1/1 -> R/1
  Divide/1 -> C/1
  Subsystem6/1(dCcoef) -> Integrator6/1
  Integrator6/1 -> Math Function/1
  Icorrect/1 -> Subsystem6/3(Icorrect)
  Cnom/1 -> Divide/1
  Urerror/1 -> Subsystem/2(Uerror)
  Subsystem/1(dRcoef) -> Integrator3/1
  Integrator3/1 -> Math Function1/1
  VTweight/1 -> Subsystem6/2(VTweight)
  Math Function/1 -> Divide/2
  Math Function1/1 -> Divide1/2

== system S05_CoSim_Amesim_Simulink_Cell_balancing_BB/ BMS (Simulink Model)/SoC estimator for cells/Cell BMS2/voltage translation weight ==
  I : Inport
  1-D Lookup Table : Lookup_n-D  NumberOfTableDimensions=1  BreakpointsForDimension1=[-0.6,-0.5,-0.1,0,0.1,0.5,0.6]  Table=[0,0,0.2,1,0.2,0,0]  InternalRulePriority=Speed  RndMeth=Simplest
  Add3 : Sum
  Gain2 : Gain  Gain=1/42
  Gain3 : Gain  Gain=0.5
  Transfer Fcn1 : TransferFcn  Denominator=[20*20*20 3*20*20 3*20 1]
  abs : Fcn  Expr=abs(u(1))
  VTweight : Outport
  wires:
  abs/1 -> Transfer Fcn1/1, Add3/1
  Gain2/1 -> abs/1  "Crate"
  Transfer Fcn1/1 -> Add3/2
  Add3/1 -> Gain3/1
  Gain3/1 -> 1-D Lookup Table/1
  I/1 -> Gain2/1
  1-D Lookup Table/1 -> VTweight/1

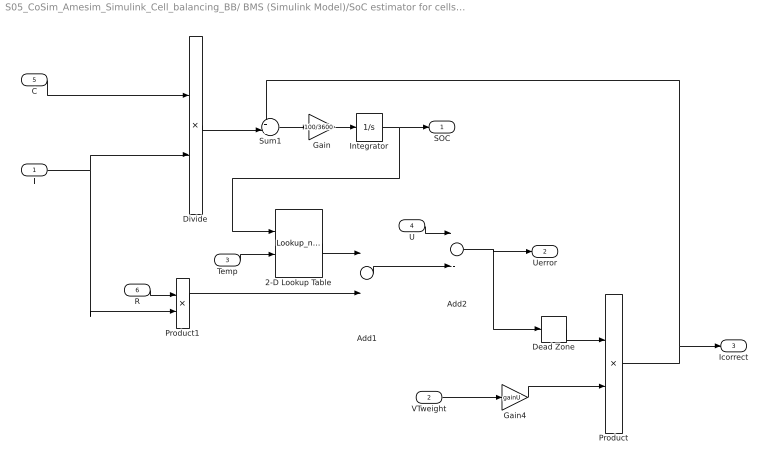
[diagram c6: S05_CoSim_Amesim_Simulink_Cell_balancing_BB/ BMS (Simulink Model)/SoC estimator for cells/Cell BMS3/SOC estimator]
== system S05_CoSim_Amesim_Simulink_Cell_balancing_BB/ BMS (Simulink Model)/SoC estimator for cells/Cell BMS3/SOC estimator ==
  I : Inport
  VTweight : Inport  Port=2
  Temp : Inport  Port=3
  U : Inport  Port=4
  C : Inport  Port=5
  R : Inport  Port=6
  2-D Lookup Table : Lookup_n-D  BreakpointsForDimension1=[0, 5, 10, 15, 20, 25, 30, 35, 40, 45, 50, 55, 60, 65, 70, 75, 80, 85, 90, 95, 100]  BreakpointsForDimension2=[0.00, 23.00, 40.00]  Table=[3.00912, 3.025112, 3.036932; 3.332236, 3.339581, 3.34501; 3.459481, 3.463587, 3.466622; 3.495249, 3.49837, 3.500677; 3.531047, 3.53332, 3.535; 3.560502, 3.562569, 3.564097; 3.588662, 3.589579, 3.590256; 3.62715, 3.625996, 3.625143; 3.648255, 3.64543, 3.643341; 3.66652, 3.663455, 3.66119; 3.685242, 3.681938, 3.679495; 3.70967, 3.706246, 3.703715; 3.738426, 3.735163, 3.732751; 3.780458, 3.777286, 3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  InternalRulePriority=Speed  RndMeth=Simplest
  Add1 : Sum
  Add2 : Sum  Inputs=+-
  Dead Zone : DeadZone  LowerValue=-0.005  UpperValue=0.005
  Divide : Product  Inputs=/*
  Gain : Gain  Gain=100/3600
  Gain4 : Gain  Gain=gainU
  Integrator : Integrator  InitialCondition=SOC_init
  Product : Product
  Product1 : Product
  Sum1 : Sum  Inputs=++|
  SOC : Outport
  Uerror : Outport  Port=2
  Icorrect : Outport  Port=3
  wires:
  Integrator/1 -> SOC/1, 2-D Lookup Table/1
  Gain/1 -> Integrator/1
  Sum1/1 -> Gain/1
  Add2/1 -> Uerror/1, Dead Zone/1
  Temp/1 -> 2-D Lookup Table/2
  C/1 -> Divide/1
  Divide/1 -> Sum1/2
  Gain4/1 -> Product/2
  R/1 -> Product1/1
  2-D Lookup Table/1 -> Add1/1
  Add1/1 -> Add2/2
  U/1 -> Add2/1
  Product1/1 -> Add1/2
  I/1 -> Divide/2, Product1/2
  Dead Zone/1 -> Product/1
  Product/1 -> Icorrect/1, Sum1/1
  VTweight/1 -> Gain4/1

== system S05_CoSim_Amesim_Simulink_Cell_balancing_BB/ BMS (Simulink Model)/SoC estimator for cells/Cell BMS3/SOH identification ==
  I : Inport
  VTweight : Inport  Port=2
  Urerror : Inport  Port=3
  Icorrect : Inport  Port=4
  Cnom : Constant  Value=42
  Divide : Product  Inputs=**
  Divide1 : Product  Inputs=**
  Integrator3 : Integrator
  Integrator6 : Integrator
  Math Function : Math
  Math Function1 : Math
  Rnom : Constant  Value=0.0022
  Subsystem : Subsystem
  Subsystem6 : Subsystem
  C : Outport
  R : Outport  Port=2
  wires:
  I/1 -> Subsystem6/1(I), Subsystem/1(I)
  Rnom/1 -> Divide1/1
  Divide1/1 -> R/1
  Divide/1 -> C/1
  Subsystem6/1(dCcoef) -> Integrator6/1
  Integrator6/1 -> Math Function/1
  Icorrect/1 -> Subsystem6/3(Icorrect)
  Cnom/1 -> Divide/1
  Urerror/1 -> Subsystem/2(Uerror)
  Subsystem/1(dRcoef) -> Integrator3/1
  Integrator3/1 -> Math Function1/1
  VTweight/1 -> Subsystem6/2(VTweight)
  Math Function/1 -> Divide/2
  Math Function1/1 -> Divide1/2

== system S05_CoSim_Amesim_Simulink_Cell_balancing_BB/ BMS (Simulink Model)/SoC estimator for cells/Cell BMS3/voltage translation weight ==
  I : Inport
  1-D Lookup Table : Lookup_n-D  NumberOfTableDimensions=1  BreakpointsForDimension1=[-0.6,-0.5,-0.1,0,0.1,0.5,0.6]  Table=[0,0,0.2,1,0.2,0,0]  InternalRulePriority=Speed  RndMeth=Simplest
  Add3 : Sum
  Gain2 : Gain  Gain=1/42
  Gain3 : Gain  Gain=0.5
  Transfer Fcn1 : TransferFcn  Denominator=[20*20*20 3*20*20 3*20 1]
  abs : Fcn  Expr=abs(u(1))
  VTweight : Outport
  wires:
  abs/1 -> Transfer Fcn1/1, Add3/1
  Gain2/1 -> abs/1  "Crate"
  Transfer Fcn1/1 -> Add3/2
  Add3/1 -> Gain3/1
  Gain3/1 -> 1-D Lookup Table/1
  I/1 -> Gain2/1
  1-D Lookup Table/1 -> VTweight/1

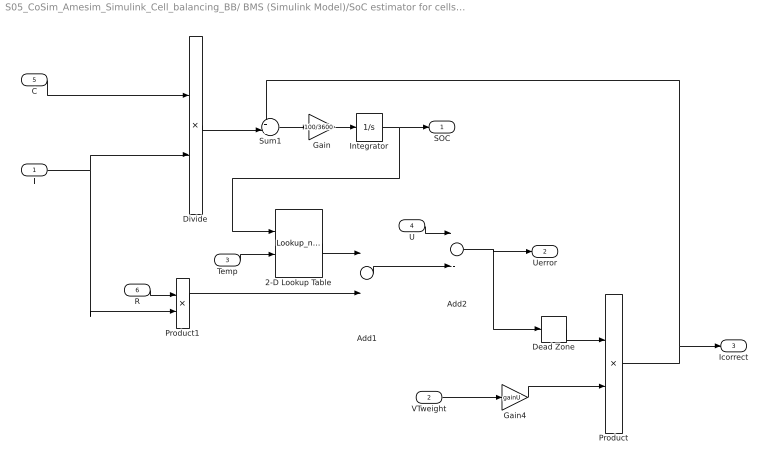
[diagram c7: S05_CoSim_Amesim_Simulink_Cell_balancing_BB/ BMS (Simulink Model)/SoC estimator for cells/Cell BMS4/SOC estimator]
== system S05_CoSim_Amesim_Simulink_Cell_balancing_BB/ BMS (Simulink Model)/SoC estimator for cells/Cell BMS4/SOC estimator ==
  I : Inport
  VTweight : Inport  Port=2
  Temp : Inport  Port=3
  U : Inport  Port=4
  C : Inport  Port=5
  R : Inport  Port=6
  2-D Lookup Table : Lookup_n-D  BreakpointsForDimension1=[0, 5, 10, 15, 20, 25, 30, 35, 40, 45, 50, 55, 60, 65, 70, 75, 80, 85, 90, 95, 100]  BreakpointsForDimension2=[0.00, 23.00, 40.00]  Table=[3.00912, 3.025112, 3.036932; 3.332236, 3.339581, 3.34501; 3.459481, 3.463587, 3.466622; 3.495249, 3.49837, 3.500677; 3.531047, 3.53332, 3.535; 3.560502, 3.562569, 3.564097; 3.588662, 3.589579, 3.590256; 3.62715, 3.625996, 3.625143; 3.648255, 3.64543, 3.643341; 3.66652, 3.663455, 3.66119; 3.685242, 3.681938, 3.679495; 3.70967, 3.706246, 3.703715; 3.738426, 3.735163, 3.732751; 3.780458, 3.777286, 3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  InternalRulePriority=Speed  RndMeth=Simplest
  Add1 : Sum
  Add2 : Sum  Inputs=+-
  Dead Zone : DeadZone  LowerValue=-0.005  UpperValue=0.005
  Divide : Product  Inputs=/*
  Gain : Gain  Gain=100/3600
  Gain4 : Gain  Gain=gainU
  Integrator : Integrator  InitialCondition=SOC_init
  Product : Product
  Product1 : Product
  Sum1 : Sum  Inputs=++|
  SOC : Outport
  Uerror : Outport  Port=2
  Icorrect : Outport  Port=3
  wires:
  Integrator/1 -> SOC/1, 2-D Lookup Table/1
  Gain/1 -> Integrator/1
  Sum1/1 -> Gain/1
  Add2/1 -> Uerror/1, Dead Zone/1
  Temp/1 -> 2-D Lookup Table/2
  C/1 -> Divide/1
  Divide/1 -> Sum1/2
  Gain4/1 -> Product/2
  R/1 -> Product1/1
  2-D Lookup Table/1 -> Add1/1
  Add1/1 -> Add2/2
  U/1 -> Add2/1
  Product1/1 -> Add1/2
  I/1 -> Divide/2, Product1/2
  Dead Zone/1 -> Product/1
  Product/1 -> Icorrect/1, Sum1/1
  VTweight/1 -> Gain4/1

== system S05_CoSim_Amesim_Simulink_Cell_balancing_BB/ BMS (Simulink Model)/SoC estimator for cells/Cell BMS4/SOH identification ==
  I : Inport
  VTweight : Inport  Port=2
  Urerror : Inport  Port=3
  Icorrect : Inport  Port=4
  Cnom : Constant  Value=42
  Divide : Product  Inputs=**
  Divide1 : Product  Inputs=**
  Integrator3 : Integrator
  Integrator6 : Integrator
  Math Function : Math
  Math Function1 : Math
  Rnom : Constant  Value=0.0022
  Subsystem : Subsystem
  Subsystem6 : Subsystem
  C : Outport
  R : Outport  Port=2
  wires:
  I/1 -> Subsystem6/1(I), Subsystem/1(I)
  Rnom/1 -> Divide1/1
  Divide1/1 -> R/1
  Divide/1 -> C/1
  Subsystem6/1(dCcoef) -> Integrator6/1
  Integrator6/1 -> Math Function/1
  Icorrect/1 -> Subsystem6/3(Icorrect)
  Cnom/1 -> Divide/1
  Urerror/1 -> Subsystem/2(Uerror)
  Subsystem/1(dRcoef) -> Integrator3/1
  Integrator3/1 -> Math Function1/1
  VTweight/1 -> Subsystem6/2(VTweight)
  Math Function/1 -> Divide/2
  Math Function1/1 -> Divide1/2

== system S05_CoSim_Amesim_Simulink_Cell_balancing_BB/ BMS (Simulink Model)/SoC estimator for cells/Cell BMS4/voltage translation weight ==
  I : Inport
  1-D Lookup Table : Lookup_n-D  NumberOfTableDimensions=1  BreakpointsForDimension1=[-0.6,-0.5,-0.1,0,0.1,0.5,0.6]  Table=[0,0,0.2,1,0.2,0,0]  InternalRulePriority=Speed  RndMeth=Simplest
  Add3 : Sum
  Gain2 : Gain  Gain=1/42
  Gain3 : Gain  Gain=0.5
  Transfer Fcn1 : TransferFcn  Denominator=[20*20*20 3*20*20 3*20 1]
  abs : Fcn  Expr=abs(u(1))
  VTweight : Outport
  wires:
  abs/1 -> Transfer Fcn1/1, Add3/1
  Gain2/1 -> abs/1  "Crate"
  Transfer Fcn1/1 -> Add3/2
  Add3/1 -> Gain3/1
  Gain3/1 -> 1-D Lookup Table/1
  I/1 -> Gain2/1
  1-D Lookup Table/1 -> VTweight/1

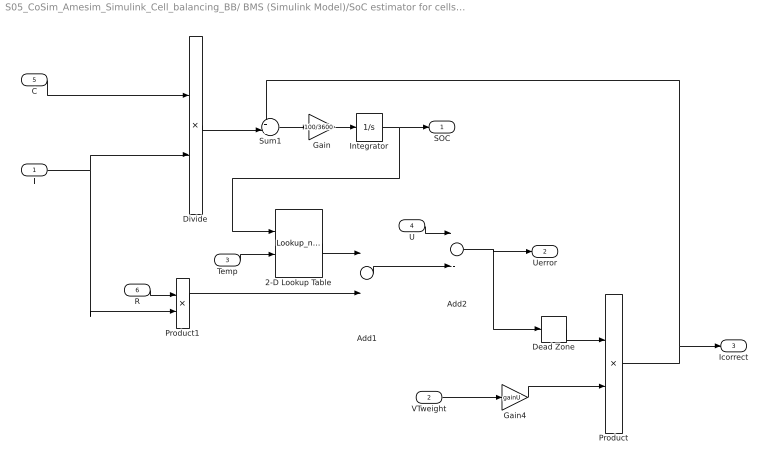
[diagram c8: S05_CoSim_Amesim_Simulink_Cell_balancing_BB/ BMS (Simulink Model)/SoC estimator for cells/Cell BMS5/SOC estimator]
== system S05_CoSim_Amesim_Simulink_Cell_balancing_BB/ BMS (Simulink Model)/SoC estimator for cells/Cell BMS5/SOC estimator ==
  I : Inport
  VTweight : Inport  Port=2
  Temp : Inport  Port=3
  U : Inport  Port=4
  C : Inport  Port=5
  R : Inport  Port=6
  2-D Lookup Table : Lookup_n-D  BreakpointsForDimension1=[0, 5, 10, 15, 20, 25, 30, 35, 40, 45, 50, 55, 60, 65, 70, 75, 80, 85, 90, 95, 100]  BreakpointsForDimension2=[0.00, 23.00, 40.00]  Table=[3.00912, 3.025112, 3.036932; 3.332236, 3.339581, 3.34501; 3.459481, 3.463587, 3.466622; 3.495249, 3.49837, 3.500677; 3.531047, 3.53332, 3.535; 3.560502, 3.562569, 3.564097; 3.588662, 3.589579, 3.590256; 3.62715, 3.625996, 3.625143; 3.648255, 3.64543, 3.643341; 3.66652, 3.663455, 3.66119; 3.685242, 3.681938, 3.679495; 3.70967, 3.706246, 3.703715; 3.738426, 3.735163, 3.732751; 3.780458, 3.777286, 3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  InternalRulePriority=Speed  RndMeth=Simplest
  Add1 : Sum
  Add2 : Sum  Inputs=+-
  Dead Zone : DeadZone  LowerValue=-0.005  UpperValue=0.005
  Divide : Product  Inputs=/*
  Gain : Gain  Gain=100/3600
  Gain4 : Gain  Gain=gainU
  Integrator : Integrator  InitialCondition=SOC_init
  Product : Product
  Product1 : Product
  Sum1 : Sum  Inputs=++|
  SOC : Outport
  Uerror : Outport  Port=2
  Icorrect : Outport  Port=3
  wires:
  Integrator/1 -> SOC/1, 2-D Lookup Table/1
  Gain/1 -> Integrator/1
  Sum1/1 -> Gain/1
  Add2/1 -> Uerror/1, Dead Zone/1
  Temp/1 -> 2-D Lookup Table/2
  C/1 -> Divide/1
  Divide/1 -> Sum1/2
  Gain4/1 -> Product/2
  R/1 -> Product1/1
  2-D Lookup Table/1 -> Add1/1
  Add1/1 -> Add2/2
  U/1 -> Add2/1
  Product1/1 -> Add1/2
  I/1 -> Divide/2, Product1/2
  Dead Zone/1 -> Product/1
  Product/1 -> Icorrect/1, Sum1/1
  VTweight/1 -> Gain4/1

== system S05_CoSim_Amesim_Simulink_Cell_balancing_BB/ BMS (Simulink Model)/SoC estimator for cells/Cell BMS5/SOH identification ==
  I : Inport
  VTweight : Inport  Port=2
  Urerror : Inport  Port=3
  Icorrect : Inport  Port=4
  Cnom : Constant  Value=42
  Divide : Product  Inputs=**
  Divide1 : Product  Inputs=**
  Integrator3 : Integrator
  Integrator6 : Integrator
  Math Function : Math
  Math Function1 : Math
  Rnom : Constant  Value=0.0022
  Subsystem : Subsystem
  Subsystem6 : Subsystem
  C : Outport
  R : Outport  Port=2
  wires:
  I/1 -> Subsystem6/1(I), Subsystem/1(I)
  Rnom/1 -> Divide1/1
  Divide1/1 -> R/1
  Divide/1 -> C/1
  Subsystem6/1(dCcoef) -> Integrator6/1
  Integrator6/1 -> Math Function/1
  Icorrect/1 -> Subsystem6/3(Icorrect)
  Cnom/1 -> Divide/1
  Urerror/1 -> Subsystem/2(Uerror)
  Subsystem/1(dRcoef) -> Integrator3/1
  Integrator3/1 -> Math Function1/1
  VTweight/1 -> Subsystem6/2(VTweight)
  Math Function/1 -> Divide/2
  Math Function1/1 -> Divide1/2

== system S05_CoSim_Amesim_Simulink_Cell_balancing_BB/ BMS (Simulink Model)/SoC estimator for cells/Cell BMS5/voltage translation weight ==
  I : Inport
  1-D Lookup Table : Lookup_n-D  NumberOfTableDimensions=1  BreakpointsForDimension1=[-0.6,-0.5,-0.1,0,0.1,0.5,0.6]  Table=[0,0,0.2,1,0.2,0,0]  InternalRulePriority=Speed  RndMeth=Simplest
  Add3 : Sum
  Gain2 : Gain  Gain=1/42
  Gain3 : Gain  Gain=0.5
  Transfer Fcn1 : TransferFcn  Denominator=[20*20*20 3*20*20 3*20 1]
  abs : Fcn  Expr=abs(u(1))
  VTweight : Outport
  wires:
  abs/1 -> Transfer Fcn1/1, Add3/1
  Gain2/1 -> abs/1  "Crate"
  Transfer Fcn1/1 -> Add3/2
  Add3/1 -> Gain3/1
  Gain3/1 -> 1-D Lookup Table/1
  I/1 -> Gain2/1
  1-D Lookup Table/1 -> VTweight/1
